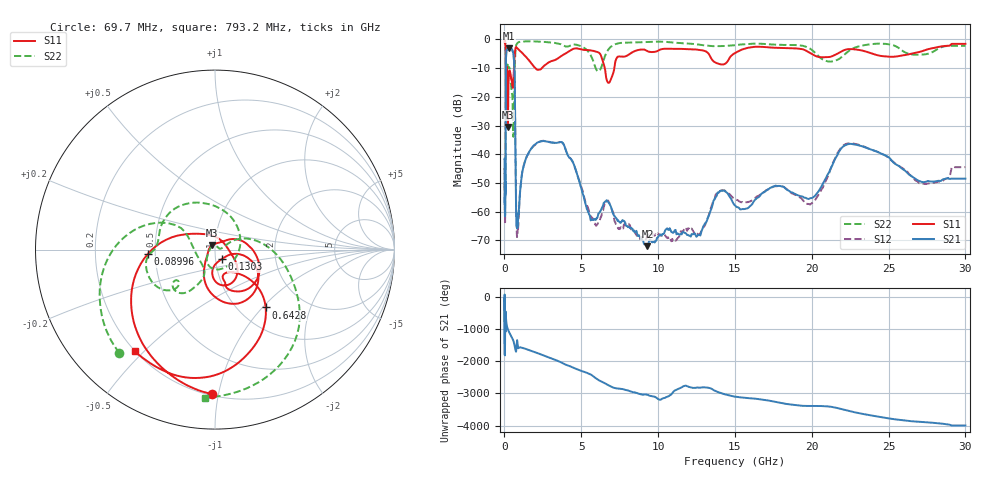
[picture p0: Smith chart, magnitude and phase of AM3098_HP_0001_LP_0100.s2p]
! Date/Time: Thu, Feb 28, 2019 8:31 AM
! Network Analyzer: Agilent Technologies E8364B Rev: A.07.50.67
! Sweep from 0.010 to 30.000 GHz, 1601 Points, Sweep Type: LOG
! Power Supply: 5.023 V, 0.002 A
# Hz S DB R 50
!freq MagS11 AngS11 MagS21 AngS21 MagS12 AngS12 MagS22 AngS22
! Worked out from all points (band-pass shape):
!   1601 points, 10 MHz to 30 GHz, reference 50 ohm
!   highest |S21| = -3.03 dB at 265.1 MHz (marker M1); lowest = -72.0 dB at 9.302 GHz (marker M2)
!   |S21| within 3 dB of the highest: 104.5 MHz to 601.5 MHz (497 MHz wide, 141 % of centre)
!   lowest |S11| = -30.5 dB at 227 MHz (marker M3), VSWR 1.06, Z = 48.1 + j2.2 ohm
!   |S11| at or under -10 dB: 176.2 MHz to 619 MHz (442.8 MHz wide, 111 % of centre); 2.013 GHz to 2.431 GHz (417.7 MHz wide, 18.8 % of centre); 6.531 GHz to 7.15 GHz (619.2 MHz wide, 9.05 % of centre)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
!   |S22| runs from -33.9 to -0.6 dB; largest |S21 - S12| = 0.013
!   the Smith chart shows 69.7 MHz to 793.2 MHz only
!   S11 on the Smith chart (normalised r, x): 69.7 MHz: 0.21, -0.96; 89.96 MHz: 0.45, -0.03; 130.3 MHz: 1.07, -0.11; 642.8 MHz: 1.32, -1.04; 793.2 MHz: 0.20, -0.47
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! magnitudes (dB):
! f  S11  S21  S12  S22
! 10 MHz  -0.4  -41.6  -46.8  -0.6
! 38.04 MHz  -0.5  -59.5  -61.0  -0.9
! 69.7 MHz  -1.9  -49.9  -51.8  -2.1
! 89.96 MHz  -8.5  -18.1  -18.0  -10.5
! 98.93 MHz  -24.2  -7.8  -7.7  -17.1
! 130.3 MHz  -23.8  -3.9  -3.9  -11.3
! 144.7 MHz  -13.4  -3.6  -3.5  -10.1
! 186.8 MHz  -11.4  -3.5  -3.4  -8.1
! 227 MHz  -30.5  -3.1  -3.1  -9.6
! 265.1 MHz  -14.8  -3.0  -3.0  -9.9
! 550.5 MHz  -16.8  -4.4  -4.3  -29.9
! 642.8 MHz  -7.4  -9.8  -9.7  -16.4
! 793.2 MHz  -2.8  -64.8  -66.0  -1.6
! 2.084 GHz  -10.4  -36.2  -36.1  -0.7
! 3.76 GHz  -5.6  -35.9  -35.9  -1.9
! 5.64 GHz  -3.8  -62.8  -61.7  -5.8
! 6.821 GHz  -15.0  -57.1  -56.9  -3.1
! 7.926 GHz  -5.8  -65.0  -64.2  -1.1
! 9.302 GHz  -4.1  -72.0  -68.3  -0.9
! 19.9 GHz  -4.8  -55.3  -57.5  -3.2
! 22.67 GHz  -3.4  -36.5  -36.2  -3.2
! 30 GHz  -1.5  -48.5  -44.5  -2.2
